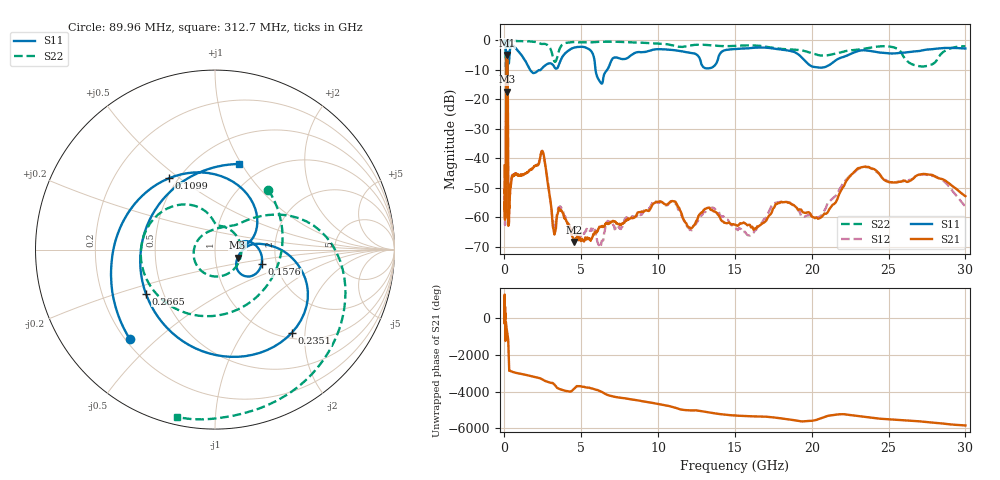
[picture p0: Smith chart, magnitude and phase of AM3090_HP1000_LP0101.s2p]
! Date/Time: Thu, Feb 28, 2019 2:02 PM
! Network Analyzer: Agilent Technologies E8364B Rev: A.07.50.67
! Sweep from 0.010 to 30.000 GHz, 1601 Points, Sweep Type: LOG
! Power Supply: 5.023 V, 0.002 A
# Hz S DB R 50
!freq MagS11 AngS11 MagS21 AngS21 MagS12 AngS12 MagS22 AngS22
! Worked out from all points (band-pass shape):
!   1601 points, 10 MHz to 30 GHz, reference 50 ohm
!   highest |S21| = -5.04 dB at 157.6 MHz (marker M1); lowest = -68.4 dB at 4.525 GHz (marker M2)
!   |S21| within 3 dB of the highest: 122.1 MHz to 204.6 MHz (82.48 MHz wide, 50.5 % of centre)
!   lowest |S11| = -17.5 dB at 191.5 MHz (marker M3), VSWR 1.31, Z = 64.1 - j5.87 ohm
!   |S11| at or under -10 dB: 119.2 MHz to 211.8 MHz (92.56 MHz wide, 55.9 % of centre); 1.656 GHz to 2.378 GHz (721.4 MHz wide, 35.8 % of centre); 5.925 GHz to 6.696 GHz (770.4 MHz wide, 12.2 % of centre)
!   |S22| runs from -19.5 to -0.2 dB; largest |S21 - S12| = 0.013
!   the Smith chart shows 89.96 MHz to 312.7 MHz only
!   S11 on the Smith chart (normalised r, x): 89.96 MHz: 0.22, -0.41; 109.9 MHz: 0.45, +0.46; 157.6 MHz: 1.67, -0.29; 235.1 MHz: 1.11, -1.71; 266.5 MHz: 0.40, -0.25; 312.7 MHz: 0.77, +0.97
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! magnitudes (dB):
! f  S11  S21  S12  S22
! 10 MHz  -0.2  -42.5  -43.7  -0.5
! 38.04 MHz  -0.5  -60.2  -60.2  -1.4
! 89.96 MHz  -3.2  -45.9  -47.2  -7.0
! 109.9 MHz  -6.5  -18.3  -18.3  -7.7
! 144.7 MHz  -12.8  -5.2  -5.1  -17.0
! 157.6 MHz  -11.3  -5.0  -5.0  -16.4
! 191.5 MHz  -17.5  -6.1  -6.1  -19.4
! 214.9 MHz  -9.0  -12.7  -12.7  -11.5
! 235.1 MHz  -4.0  -39.5  -39.6  -2.7
! 250.9 MHz  -4.9  -61.0  -58.1  -1.3
! 266.5 MHz  -6.8  -59.3  -60.6  -0.8
! 312.7 MHz  -6.1  -56.7  -56.9  -0.4
! 550.5 MHz  -2.0  -45.9  -45.7  -0.2
! 2.084 GHz  -10.8  -42.5  -42.3  -0.7
! 2.507 GHz  -9.3  -38.0  -38.0  -1.3
! 3.22 GHz  -8.9  -65.1  -63.4  -6.9
! 4.525 GHz  -2.6  -68.4  -65.5  -0.7
! 6.234 GHz  -14.2  -63.3  -69.3  -0.6
! 7.926 GHz  -6.3  -60.9  -60.1  -0.7
! 15.97 GHz  -2.8  -62.6  -66.3  -1.8
! 23.48 GHz  -3.5  -42.9  -43.0  -2.9
! 30 GHz  -2.9  -52.9  -56.4  -2.1
